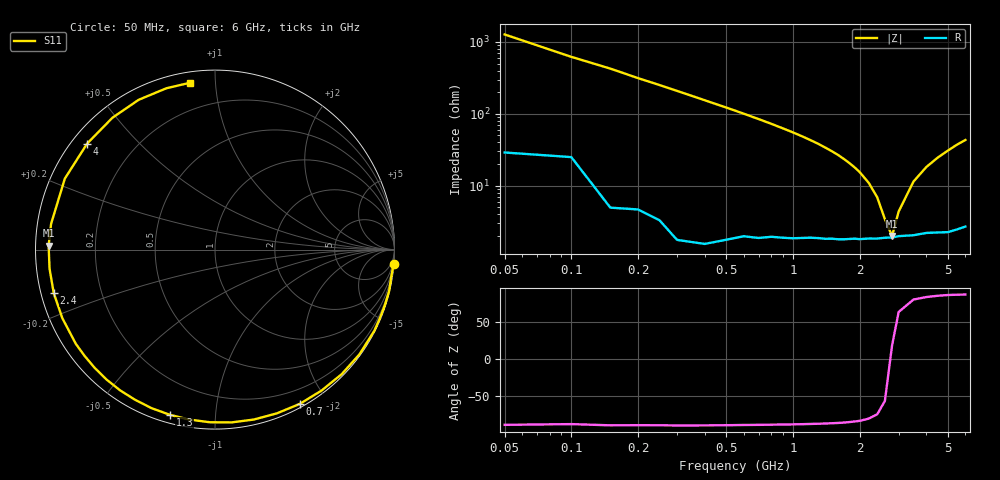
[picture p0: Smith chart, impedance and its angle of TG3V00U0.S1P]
! SIEMENS Discrete & RF Semiconductors
! BAT64
! Si Schottky Diode in SOT23
! VR = 3 V
! S-Parameters:  February  1997
# GHz  S  MA  R  50
!  f  S11
! GHz  MAG  ANG
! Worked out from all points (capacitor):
!   34 points, 50 MHz to 6 GHz, reference 50 ohm
!   read as one part to ground: C = 2.5 pF near 50 MHz
!   lowest |Z| = 1.99 ohm at 2.8 GHz (marker M1)
!   series resonance near 2.765 GHz, so ESL is about 1.3 nH
!   S11 on the Smith chart (normalised r, x): 50 MHz: 1, -25; 700 MHz: 0.04, -1.69; 1.3 GHz: 0.04, -0.76; 2.4 GHz: 0.04, -0.13; 4 GHz: 0.04, +0.36; 6 GHz: 0.05, +0.86
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0.05  0.9982 -4.5
0.15  0.9973 -13.4
0.3  0.9962 -27.0
0.4  0.9942 -35.9
0.5  0.9899 -44.5
0.6  0.9844 -53.0
0.7  0.9808 -61.3
0.8  0.9753 -69.3
0.9  0.9712 -77.1
1  0.9672 -84.5
1.1  0.9623 -91.7
1.2  0.9577 -98.7
1.3  0.9541 -105.3
1.4  0.9514 -111.9
1.6  0.9457 -124.0
1.8  0.94 -135.5
2  0.9365 -145.9
2.2  0.9324 -155.8
2.4  0.9306 -164.9
2.6  0.9279 -173.5
2.8  0.9272 178.6
3  0.9244 171.1
3.5  0.9254 154.7
4  0.9254 140.3
4.5  0.9307 127.9
5  0.9367 117.0
5.5  0.9388 106.8
6  0.9402 98.4
